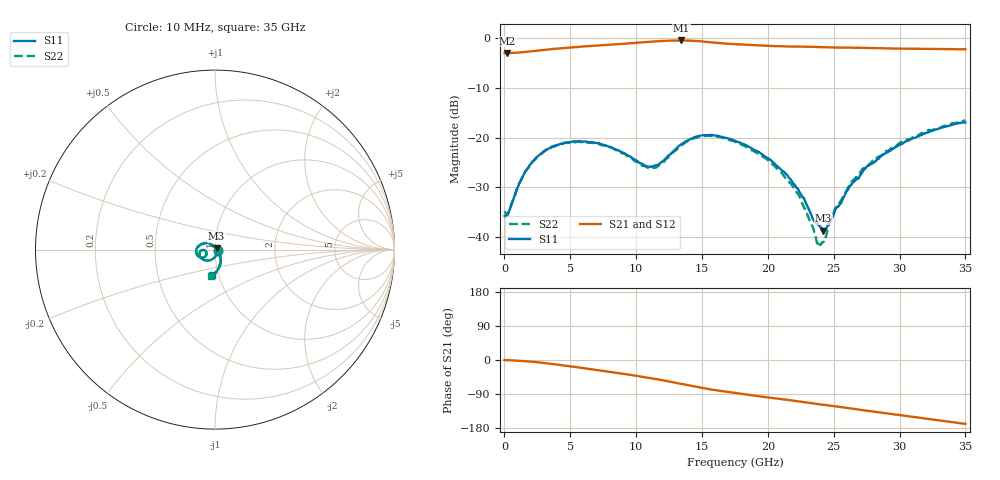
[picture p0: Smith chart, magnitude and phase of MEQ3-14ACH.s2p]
! MARKI MICROWAVE INC.
! Email:  support@markimicrowave.com  Phone:  408-778-4200
! Model Number:  MEQ3-14ACH  Date:  6/18
! Filename:		MEQ3-14ACH.S2P  Version: 1.0
! Description:  2-port S-parameter data for chip equalizer
! Features:		Low Insertion Loss, Excellent Return Loss
! Frequency Measured: 	10 MHz to 35 GHz
!S2P File: Measurements: S11, S21, S12, S22:
# Hz S  dB  R 50
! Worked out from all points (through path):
!   1601 points, 10 MHz to 35 GHz, reference 50 ohm
!   highest |S21| = -0.47 dB at 13.44 GHz (marker M1); lowest = -3.0 dB at 206.8 MHz (marker M2)
!   group delay of S21, straight-line fit = 14.1 ps
!   lowest |S11| = -38.7 dB at 24.22 GHz (marker M3), VSWR 1.02, Z = 50.9 + j0.745 ohm
!   |S11| at or under -10 dB: start of sweep to end of sweep
!   |S22| runs from -41.8 to -16.5 dB; largest |S21 - S12| = 0.0077
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1e7  -35.72 -25.0  -2.99 -0.1  -3.06 0.1  -34.77 -5.0
2.068188e8  -35.64 -23.4  -3.01 -0.3  -3.01 -0.4  -35.49 -24.5
1.343994e9  -27.95 -88.5  -2.84 -2.6  -2.84 -2.6  -28.13 -88.6
2.393694e9  -24.02 -112.5  -2.55 -5.6  -2.55 -5.6  -24.18 -113.1
4.077588e9  -21.44 -138.3  -2.08 -12.4  -2.09 -12.4  -21.33 -138.6
5.848956e9  -20.74 -158.1  -1.70 -20.7  -1.71 -20.7  -20.92 -157.9
8.145175e9  -21.95 -175.4  -1.30 -31.9  -1.30 -31.9  -21.98 -175.4
1.090064e10  -25.76 -166.2  -0.76 -46.6  -0.76 -46.6  -26.08 -166.4
1.168791e10  -25.40 -153.4  -0.63 -51.4  -0.62 -51.4  -25.59 -152.8
1.343741e10  -21.34 -148.4  -0.47 -63.1  -0.47 -63.2  -21.53 -147.3
1.533999e10  -19.50 -169.6  -0.76 -75.7  -0.76 -75.6  -19.61 -168.5
1.7505e10  -20.62 166.5  -1.21 -86.8  -1.22 -87.0  -20.81 167.4
2.1004e10  -26.43 133.7  -1.63 -103.1  -1.61 -103.3  -26.91 136.2
2.231612e10  -30.48 118.4  -1.71 -109.1  -1.74 -109.2  -31.40 119.8
2.334396e10  -35.89 93.5  -1.76 -114.1  -1.75 -113.9  -37.59 92.8
2.382507e10  -37.35 66.1  -1.80 -116.4  -1.76 -116.2  -41.57 62.1
2.421871e10  -38.69 39.0  -1.83 -118.3  -1.77 -118.2  -40.87 17.8
2.511532e10  -34.40 -18.5  -1.88 -122.3  -1.84 -122.5  -34.26 -28.7
2.633998e10  -29.32 -39.6  -1.93 -128.0  -1.95 -128.2  -28.83 -46.5
2.918291e10  -22.75 -65.0  -2.09 -141.4  -2.04 -141.6  -22.60 -67.0
3.189464e10  -19.16 -80.7  -2.15 -154.1  -2.16 -153.8  -19.08 -81.4
3.5e10  -16.95 -95.7  -2.25 -168.5  -2.24 -168.8  -16.51 -98.0
